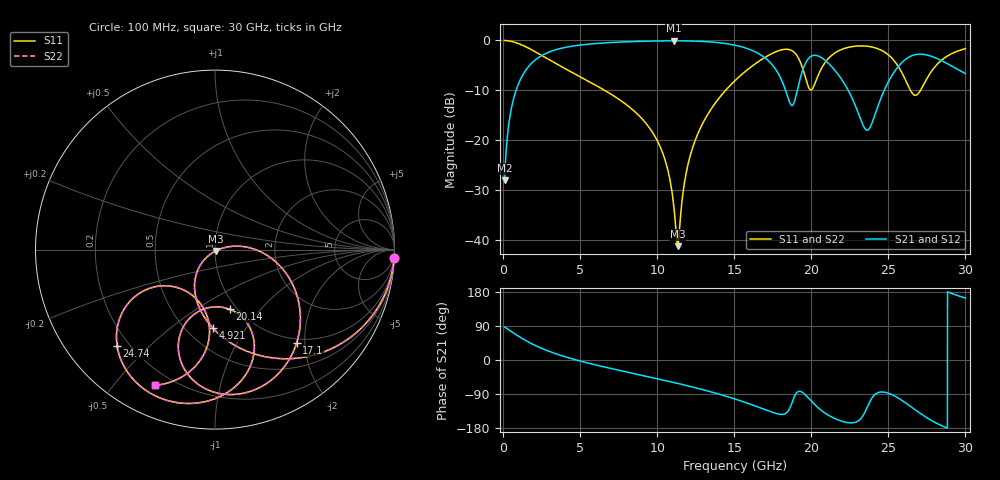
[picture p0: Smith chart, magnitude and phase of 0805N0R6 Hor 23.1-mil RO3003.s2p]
# GHz S MA R 50
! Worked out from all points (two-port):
!   3201 points, 100 MHz to 30 GHz, reference 50 ohm
!   highest |S21| = -0.08 dB at 11.09 GHz (marker M1); lowest = -28.1 dB at 100 MHz (marker M2)
!   |S21| within 3 dB of the highest: 2.485 GHz to 16.81 GHz (14.32 GHz wide, 148 % of centre); 26.51 GHz to 27.69 GHz (1.176 GHz wide, 4.34 % of centre)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
!   lowest |S11| = -41.3 dB at 11.33 GHz (marker M3), VSWR 1.02, Z = 50.4 - j0.776 ohm
!   |S11| at or under -10 dB: 6.585 GHz to 14.44 GHz (7.857 GHz wide, 74.7 % of centre); 26.43 GHz to 27.09 GHz (653.8 MHz wide, 2.44 % of centre)
!   |S22| runs from -41.3 to 0.0 dB; largest |S21 - S12| = 0
!   S11 on the Smith chart (normalised r, x): 100 MHz: 1, -40; 4.921 GHz: 0.67, -0.72; 17.1 GHz: 0.92, -1.83; 20.14 GHz: 0.93, -0.70; 24.74 GHz: 0.15, -0.40; 30 GHz: 0.13, -0.64
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0.1  0.9992 -2.8  0.03942 87.2  0.03942 87.2  0.9992 -2.8
0.5485  0.9773 -15.4  0.2115 74.6  0.2115 74.6  0.9773 -15.4
1.333375  0.8843 -35.4  0.466 54.5  0.466 54.5  0.8843 -35.4
4.921375  0.4383 -91.4  0.8953 -1.9  0.8953 -1.9  0.4383 -91.4
5.089563  0.4244 -93.2  0.9019 -3.7  0.9019 -3.7  0.4244 -93.2
10.06978  0.09433 -135.7  0.9882 -49.9  0.9882 -49.9  0.09433 -135.7
11.08825  0.0211 -126.3  0.9911 -59.4  0.9911 -59.4  0.0211 -126.3
11.33119  0.008652 -62.8  0.991 -61.7  0.991 -61.7  0.008652 -62.8
12.45244  0.09818 10.8  0.984 -72.9  0.984 -72.9  0.09818 10.8
15.05  0.3955 -16.3  0.8949 -102.9  0.8949 -102.9  0.3955 -16.3
17.09628  0.6908 -48.8  0.6493 -132.4  0.6493 -132.4  0.6908 -48.8
18.75013  0.7883 -91.8  0.2227 -112.7  0.2227 -112.7  0.7883 -91.8
19.37616  0.5603 -111.3  0.4675 -84.2  0.4675 -84.2  0.5603 -111.3
20.03956  0.323 -83.5  0.7004 -110.2  0.7004 -110.2  0.323 -83.5
20.14234  0.3424 -76.2  0.7081 -114.6  0.7081 -114.6  0.3424 -76.2
21.23556  0.6894 -73.9  0.5638 -148.6  0.5638 -148.6  0.6894 -73.9
23.5715  0.8768 -114.6  0.1264 -129.8  0.1264 -129.8  0.8768 -114.6
24.73947  0.7666 -135.3  0.3174 -84.9  0.3174 -84.9  0.7666 -135.3
25.01978  0.7127 -140.2  0.3892 -87.9  0.3892 -87.9  0.7127 -140.2
26.76706  0.2816 -121.0  0.7214 -132.2  0.7214 -132.2  0.2816 -121.0
27.93503  0.5233 -94.2  0.6803 -162.7  0.6803 -162.7  0.5233 -94.2
30  0.8272 -113.8  0.4642 163.5  0.4642 163.5  0.8272 -113.8
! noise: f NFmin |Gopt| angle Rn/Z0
0.1  0.001588  0.9683  1.525  0.01136
3.417  0.00768  0.7527  21.17  0.006059
6.743  0.01319  0.7245  38.81  0.008483
10.06  0.0196  0.7305  55.57  0.01142
13.39  0.03119  0.7765  71.43  0.01897
16.7  0.08079  0.8894  86.91  0.08404
20.03  0.1997  0.9461  101.8  0.3308
23.35  0.7371  0.983  115.5  2.836
26.67  0.2211  0.9378  128.7  0.1493
30  0.178  0.9152  140.9  0.05274
